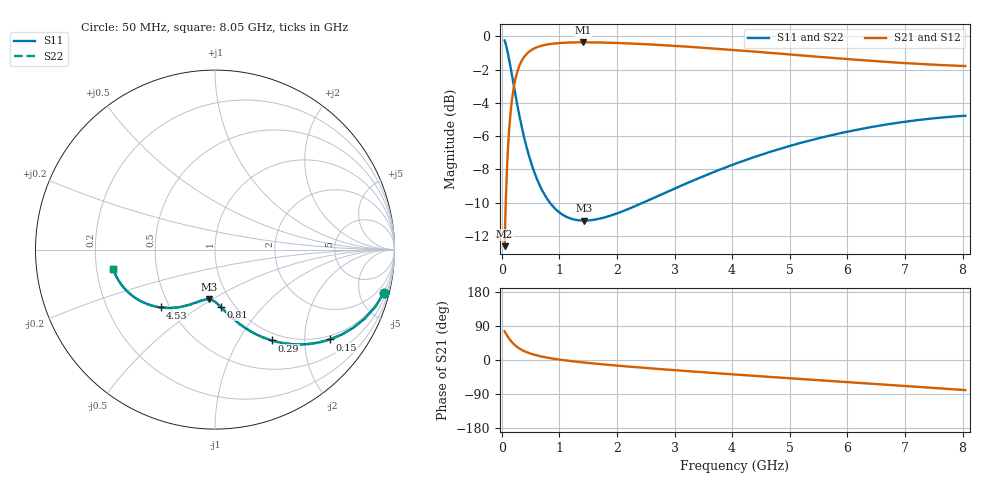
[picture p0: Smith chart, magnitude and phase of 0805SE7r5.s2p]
! AVX Thin Film Operation		Date: August 2001
! Description: Accu-P® Series, Thin Film, SMD, RF Capacitor
! Part Number: 08051J7R5BBT
! 50 MHz  -  8.05 GHz
! Serial Measurements
# mhz S db R 50
!	S11		S21		S12		S22
!	dB	Phase	dB	Phase	dB	Phase	dB	Phase
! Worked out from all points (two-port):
!   401 points, 50 MHz to 8.05 GHz, reference 50 ohm
!   highest |S21| = -0.36 dB at 1.41 GHz (marker M1); lowest = -12.6 dB at 50 MHz (marker M2)
!   |S21| within 3 dB of the highest: 196.3 MHz to end of sweep
!   lowest |S11| = -11.1 dB at 1.43 GHz (marker M3), VSWR 1.78, Z = 40.4 - j24.3 ohm
!   |S11| at or under -10 dB: 836.7 MHz to 2.453 GHz (1.617 GHz wide, 98.3 % of centre)
!   |S22| runs from -11.1 to -0.2 dB; largest |S21 - S12| = 0
!   S11 on the Smith chart (normalised r, x): 50 MHz: 0.89, -7.85; 150 MHz: 0.89, -2.64; 290 MHz: 0.89, -1.40; 810 MHz: 0.86, -0.61; 4.53 GHz: 0.45, -0.36; 8.05 GHz: 0.27, -0.09
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50  -0.24 -14.3  -12.61 75.7  -12.61 75.7  -0.24 -14.3
90  -0.74 -24.8  -8.04 65.2  -8.04 65.2  -0.74 -24.8
110  -1.07 -29.6  -6.63 60.4  -6.63 60.4  -1.07 -29.6
150  -1.79 -38.0  -4.71 52.0  -4.71 52.0  -1.79 -38.0
210  -2.97 -48.1  -3.05 41.9  -3.05 41.9  -2.97 -48.1
250  -3.74 -53.5  -2.39 36.5  -2.39 36.5  -3.74 -53.5
290  -4.48 -58.0  -1.92 32.0  -1.92 32.0  -4.48 -58.0
370  -5.79 -65.0  -1.33 24.9  -1.33 24.9  -5.79 -65.0
490  -7.37 -72.5  -0.88 17.5  -0.88 17.5  -7.37 -72.5
630  -8.72 -78.6  -0.63 11.4  -0.63 11.4  -8.72 -78.6
810  -9.87 -84.2  -0.47 5.7  -0.47 5.7  -9.87 -84.2
1070  -10.75 -90.2  -0.39 -0.3  -0.39 -0.3  -10.75 -90.2
1390  -11.07 -95.9  -0.36 -6.0  -0.36 -6.0  -11.07 -96.0
1410  -11.08 -96.3  -0.36 -6.3  -0.36 -6.3  -11.08 -96.3
1430  -11.08 -96.6  -0.36 -6.7  -0.36 -6.7  -11.08 -96.6
2010  -10.63 -104.8  -0.40 -14.9  -0.40 -14.9  -10.63 -104.8
2730  -9.57 -113.6  -0.51 -23.7  -0.51 -23.7  -9.57 -113.6
4050  -7.66 -128.2  -0.82 -38.3  -0.82 -38.3  -7.66 -128.2
4530  -7.09 -133.2  -0.95 -43.4  -0.95 -43.4  -7.09 -133.2
5390  -6.22 -142.1  -1.20 -52.2  -1.20 -52.2  -6.22 -142.1
6730  -5.27 -155.6  -1.55 -65.8  -1.55 -65.8  -5.27 -155.7
8050  -4.77 -169.2  -1.78 -79.4  -1.78 -79.4  -4.77 -169.2
